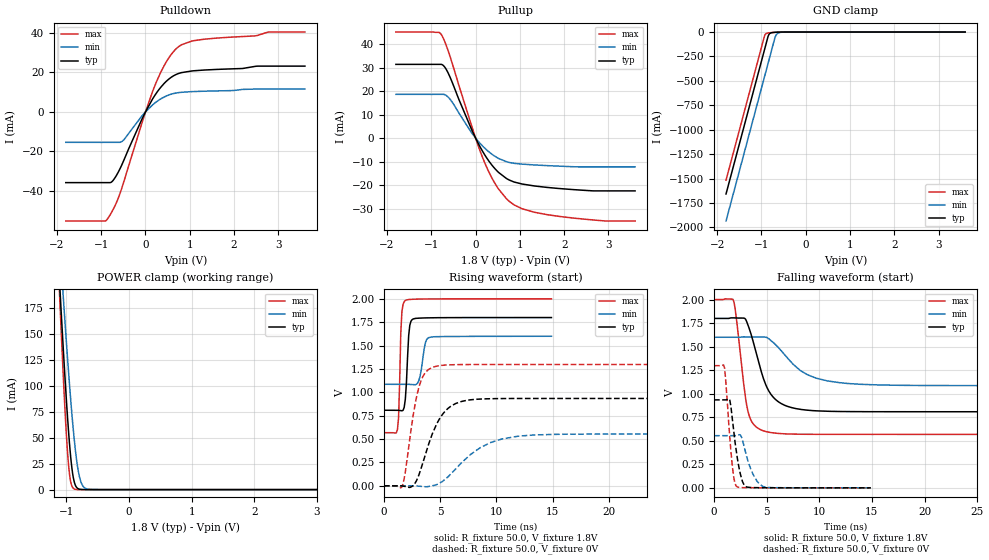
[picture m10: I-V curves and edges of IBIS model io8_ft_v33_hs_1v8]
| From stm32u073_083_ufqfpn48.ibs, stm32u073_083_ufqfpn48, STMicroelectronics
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[Model]   io8_ft_v33_hs_1v8
Model_type I/O
Polarity   Non-Inverting
Enable   Active-Low
| CAP_THRESHOLD on pad IOFT is "UDTCAPC" :
| Rising=30.0% of vddiom   Falling=70.0% of vddiom
| C_comp min and max val. don't necessarily correlate with the min and max pvt
| but are the smallest and greatest pad capacitance found.
| var   typ   min   max
C_comp   2.10717pF  2.10454pF  2.16859pF
|C_comp_pullup   1.19920pF  1.17990pF  1.18495pF
|C_comp_pulldown   907.97315fF  924.63568fF  983.64002fF
Vinl = 480.0mV
Vinh = 1.4V
Vmeas = 900.0mV   | Reference voltage for timing measurements
Cref  = 50.0pF   | Timing specification test load capacitance value
Rref  = 100.0MOhm   | Timing specification test load resistance value
Vref  = 900.0mV   | Timing specification test load voltage
[Model Spec]
| TIME_THRESHOLD on pin ZIV33M is "CMOS" :
| Rising=50.0% of vddiom   Falling=50.0% of vddiom
Vinl 728.70000mV 655.70000mV 817.70000mV
Vinh 1.06430V 949.30000mV 1.16330V
| variable   typ   min   max
[Temperature Range] 25.0 140.0 -40.0
| variable   typ   min   max
[Voltage Range] 1.8V 1.6V 2.0V
| variable   typ   min   max
[POWER Clamp Reference] 1.8V 1.6V 2.0V
| variable   typ   min   max
[GND Clamp Reference] 0V 0V 0V
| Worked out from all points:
|   slope of the pulldown table from 0 to 0.27 V, typ, clamps not added: 26.3 ohm
|   slope of the pullup table from 0 to 0.27 V, typ, clamps not added: 30 ohm
|   GND clamp passes 1 mA (typ) near -0.61 V on its own axis
|   POWER clamp passes 1 mA (typ) near -0.81 V on its own axis
|   rising waveform, R_fixture 50.0, V_fixture 1.8V: 20-80 % time 252ps typ, 394ps min, 200ps max; typ from 0.809 V to 1.8 V
|   falling waveform, R_fixture 50.0, V_fixture 1.8V: 20-80 % time 1.73ns typ, 3.11ns min, 931ps max; typ from 1.8 V to 0.809 V
|   rising waveform, R_fixture 50.0, V_fixture 0V: 20-80 % time 1.8ns typ, 3.34ns min, 1.04ns max; typ from 0 V to 0.935 V
|   falling waveform, R_fixture 50.0, V_fixture 0V: 20-80 % time 697ps typ, 1.03ns min, 537ps max; typ from 0.935 V to 0 V
[POWER Clamp]
-1.8V     1.053A     943.1mA    1.262A
-1.11V    202.2mA    242.3mA    190.9mA
-1.09V    180mA      223.6mA    163.4mA
-1.05V    136.9mA    187mA      110.9mA
-980mV    68.91mA    126.1mA    35.23mA
-940mV    37.57mA    94.11mA    10.65mA
-880mV    8.969mA    52.17mA    807.4uA
-830mV    1.697mA    25.82mA    75.79uA
-790mV    394.2uA    12.22mA    11.25uA
-740mV    61.25uA    3.879mA    1.034uA
-660mV    3.073uA    483.4uA    22.7nA
3.6V      0A         0A         0A
[GND Clamp]
-1.8V     -1.658A    -1.935A    -1.517A
-930mV    -179mA     -456mA     -38.91mA
-900mV    -128mA     -405mA     -17.65mA
-850mV    -44.09mA   -320mA     -9.519mA
-830mV    -24.74mA   -286mA     -8.302mA
-790mV    -9.695mA   -218mA     -6.49mA
-700mV    -2.938mA   -65mA      -3.294mA
-670mV    -2.157mA   -31.85mA   -2.435mA
-640mV    -1.545mA   -16.21mA   -1.699mA
-570mV    -571.9uA   -3.807mA   -536.5uA
-420mV    -14.26uA   -143.3uA   -5.434uA
3.6V      449.1pA    102.3nA    316.4pA
| variable   typ   min   max
[Pullup Reference] 1.8V 1.6V 2.0V
| variable   typ   min   max
[Pulldown Reference] 0V 0V 0V
[Pullup]
-1.8V     31.43mA    18.65mA    45.21mA
-780mV    31.43mA    18.65mA    44.28mA
-690mV    30.07mA    18.48mA    40.79mA
-580mV    26.09mA    16.61mA    34.95mA
-90mV     3.62mA     2.224mA    5.223mA
180mV     -6.337mA   -3.799mA   -9.336mA
470mV     -13.71mA   -8.14mA    -20.34mA
760mV     -17.88mA   -10.38mA   -26.96mA
1.05V     -19.57mA   -11.08mA   -30.1mA
1.62V     -21.02mA   -11.72mA   -32.63mA
2.94V     -22.49mA   -12.26mA   -35.33mA
3.6V      -22.49mA   -12.26mA   -35.33mA
[Pulldown]
-1.8V     -35.76mA   -15.41mA   -55.17mA
-910mV    -35.76mA   -15.41mA   -55.17mA
-830mV    -35.76mA   -15.41mA   -53.18mA
-710mV    -34mA      -15.41mA   -48.42mA
-520mV    -26.05mA   -14.75mA   -37.5mA
-90mV     -4.145mA   -2.306mA   -6.327mA
230mV     8.974mA    4.797mA    14.24mA
490mV     15.87mA    8.223mA    26.01mA
750mV     19.43mA    9.743mA    33.01mA
1.33V     21.16mA    10.45mA    36.75mA
2.78V     23.13mA    11.52mA    40.36mA
3.6V      23.13mA    11.52mA    40.37mA
[Ramp]
dV/dt_r 560.73574mV/1.80346ns 332.4142mV/3.33763ns 778.77819mV/1.04145ns
dV/dt_f 594.84395mV/1.72688ns 308.29327mV/3.10665ns 859.13213mV/927.30943ps
R_load = 50.0
| Removed startup time: 0s 0s 0s  .
| Removed end time: 14.9ns.
[Rising Waveform]
R_fixture   = 50.0
V_fixture   = 1.8V
V_fixture_min = 1.6V
V_fixture_max = 2.0V
0s        808.6mV    1.086V     568.1mV
1.2ns     808.4mV    1.086V     601.9mV
1.3ns     807.7mV    1.086V     727.4mV
1.5ns     804.5mV    1.086V     1.641V
1.6ns     802.6mV    1.086V     1.866V
1.9ns     924.1mV    1.086V     1.983V
2.2ns     1.607V     1.085V     1.993V
2.6ns     1.785V     1.082V     1.996V
4ns       1.797V     1.586V     1.999V
14.9ns    1.8V       1.6V       2V
| Removed startup time: 0s 0s 0s  .
| Removed end time: 39.9ns.
[Falling Waveform]
R_fixture   = 50.0
V_fixture   = 1.8V
V_fixture_min = 1.6V
V_fixture_max = 2.0V
0s        1.8V       1.6V       2V
1.8ns     1.806V     1.6V       2.002V
2ns       1.805V     1.6V       1.904V
3.2ns     1.736V     1.604V     823.4mV
3.7ns     1.56V      1.603V     682.7mV
4.7ns     1.159V     1.602V     605.5mV
6.7ns     877.6mV    1.415V     573.6mV
8.8ns     825.9mV    1.206V     569mV
11.7ns    811.3mV    1.12V      568.1mV
39.9ns    808.6mV    1.086V     568.1mV
| Removed startup time: 0s 0s 0s  .
| Removed end time: 39.9ns.
[Rising Waveform]
R_fixture   = 50.0
V_fixture   = 0V
V_fixture_min = 0V
V_fixture_max = 0V
0s        -9.618uV   -5.539uV   -9.598uV
1.6ns     -405.7uV   -519.1nV   -12.81mV
2.5ns     -5.927mV   179.2uV    676.7mV
3.1ns     113.1mV    -4.01mV    1.049V
3.7ns     342.3mV    -10.07mV   1.213V
4.6ns     637.4mV    9.76mV     1.277V
6.9ns     902.1mV    246.1mV    1.297V
9.5ns     932mV      463.5mV    1.298V
11.9ns    934.3mV    530.1mV    1.298V
39.9ns    934.6mV    554mV      1.298V
| Removed startup time: 0s 0s 0s  .
| Removed end time: 14.9ns.
[Falling Waveform]
R_fixture   = 50.0
V_fixture   = 0V
V_fixture_min = 0V
V_fixture_max = 0V
0s        934.6mV    554mV      1.298V
1ns       934.1mV    554mV      1.271V
1.5ns     929.9mV    553.8mV    524.8mV
1.7ns     771.8mV    553.7mV    271mV
1.9ns     570.9mV    554mV      91.92mV
2.2ns     322.8mV    558.9mV    10.25mV
2.9ns     24.97mV    418.6mV    1.66mV
3.7ns     2.694mV    144.5mV    791uV
4.6ns     1.108mV    15.58mV    381.6uV
14.9ns    1.657uV    36.38uV    368nV
